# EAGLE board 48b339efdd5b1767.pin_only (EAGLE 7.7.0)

Size 17.78 x 52.07 mm. Coordinates in mm from the lower left corner, seen from the top.
Outline: 0,0 0,52.07 17.78,52.07 17.78,0 0,0
Copper layers (1*16): Top 0.035mm / dielectric 1.5mm / Bottom 0.035mm
Design rules "SparkFun-2-layer-FAB-LIMIT *": minimum track width 4mil, minimum drill 6mil, track to track 6mil, track to pad 6mil, pad to pad 6mil, via to via 6mil, smd to smd 6mil, copper to edge 4mil, drill to drill 4mil, minimum pad ring 5mil, minimum via ring 5mil, stop-mask expansion 4mil, vias tented up to drill 25mil, thermal gap 10mil
tRestrict: 2 lines

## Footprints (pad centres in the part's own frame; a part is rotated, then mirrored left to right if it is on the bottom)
0603 = smd 1.1 x 1: 1 -0.85,0; 2 0.85,0
0402 = smd 0.85 x 0.9: 1 -0.58,0; 2 0.58,0
LED-0603 = smd 1 x 1: A -0.877,0; C 0.877,0
TRACE_ANTENNA_2.4GHZ_15.2MM = smd 0.5 x 0.5: ANT 0,-0.25 | smd 0.9 x 0.5: GND -2.1,-0.25
FIDUCIAL-MICRO = smd 0.635 x 0.635: 1 0,0
1X06 = drill 1.016 pad 1.88: 1 0,0; 2 2.54,0; 3 5.08,0; 4 7.62,0; 5 10.16,0; 6 12.7,0
1X02 = drill 1.016 pad 1.88: 1 0,0; 2 2.54,0
1X17 = drill 1.016 pad 1.88: 1 0,0; 2 2.54,0; 3 5.08,0; 4 7.62,0; 5 10.16,0; 6 12.7,0; 7 15.24,0; 8 17.78,0; 9 20.32,0; 10 22.86,0; 11 25.4,0; 12 27.94,0; 13 30.48,0; 14 33.02,0; 15 35.56,0; 16 38.1,0; 17 40.64,0
2X5-PTH-1.27MM = drill 0.508 pad 1: 1 -2.54,-0.635; 2 -2.54,0.635; 3 -1.27,-0.635; 4 -1.27,0.635; 5 0,-0.635; 6 0,0.635; 7 1.27,-0.635; 8 1.27,0.635; 9 2.54,-0.635; 10 2.54,0.635
SMT-JUMPER_2_NC_TRACE_SILK = smd 0.635 x 1.27: 1 -0.508,0; 2 0.508,0
SMT-JUMPER_2_NO_SILK = smd 0.635 x 1.27: 1 -0.406,0; 2 0.406,0
PAD-JUMPER-2-NC_BY_TRACE_YES_SILK = smd 0.635 x 1.27: 1 -0.508,0; 2 0.508,0
TACTILE_SWITCH_SMD_4.6X2.8MM = smd 0.9 x 1: 1 -2.05,-0.8; 2 2.05,-0.8; 3 2.05,0.8; 4 -2.05,0.8
PAD.03X.04 = smd 1.016 x 1.016: P$1 0,0
SOT23-5 = smd 0.55 x 1.2: 1 -0.95,-1.3; 2 0,-1.3; 3 0.95,-1.3; 4 0.95,1.3; 5 -0.95,1.3
QFN48-6X6MM = smd 0.68 x 0.23: 1 -2.86,2.2; 2 -2.86,1.8; 3 -2.86,1.4; 4 -2.86,1; 5 -2.86,0.6; 6 -2.86,0.2; 7 -2.86,-0.2; 8 -2.86,-0.6; 9 -2.86,-1; 10 -2.86,-1.4; 11 -2.86,-1.8; 12 -2.86,-2.2; 25 2.86,-2.2; 26 2.86,-1.8; 27 2.86,-1.4; 28 2.86,-1; 29 2.86,-0.6; 30 2.86,-0.2; 31 2.86,0.2; 32 2.86,0.6; 33 2.86,1; 34 2.86,1.4; 35 2.86,1.8; 36 2.86,2.2 | smd 0.23 x 0.68: 13 -2.2,-2.86; 14 -1.8,-2.86; 15 -1.4,-2.86; 16 -1,-2.86; 17 -0.6,-2.86; 18 -0.2,-2.86; 19 0.2,-2.86; 20 0.6,-2.86; 21 1,-2.86; 22 1.4,-2.86; 23 1.8,-2.86; 24 2.2,-2.86; 37 2.2,2.86; 38 1.8,2.86; 39 1.4,2.86; 40 1,2.86; 41 0.6,2.86; 42 0.2,2.86; 43 -0.2,2.86; 44 -0.6,2.86; 45 -1,2.86; 46 -1.4,2.86; 47 -1.8,2.86; 48 -2.2,2.86 | smd 4.6 x 4.6: EP 0,0
CRYSTAL-SMD-2.0X1.6MM = smd 0.75 x 0.7: 1 -0.675,-0.5; 2 0.675,-0.5; 3 0.675,0.5; 4 -0.675,0.5
CRYSTAL-SMD-3.2X1.5MM = smd 1 x 1.8: P$1 -1.25,0; P$2 1.25,0

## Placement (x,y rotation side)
C1  1.0uF  [0603]  5.71,6.35 270 top
C2  2.2uF  [0603]  12.06,6.35 270 top
C3  0.1uF  [0402]  6.35,30.48 90 top
C4  DNP  [0402]  7.87,41.91 270 top
C5  100pF  [0402]  6.5,41.91 270 top
C6  1.0uF  [0402]  5.08,33.66 270 top
C7  180pF  [0603]  5.71,24.13 90 top
C8  180pF  [0603]  12.7,24.13 90 top
C9  6pF  [0402]  4.45,43.18 180 top
C10  6pF  [0402]  4.45,39.47 180 top
C11  0.8pF  [0402]  9.53,40.31 0 top
C12  DNP  [0402]  9.53,44.45 180 top
C13  15pF  [0402]  8.13,29.84 180 top
C14  15pF  [0402]  10.59,29.84 0 top
C15  0.1uF  [0402]  13.97,32.77 270 top
C16  0.1uF  [0402]  4.45,38.1 180 top
C17  4.7uF  [0603]  5.08,30.48 270 top
D1  RED  [LED-0603]  6.35,16.51 0 top
D2  BLUE  [LED-0603]  11.43,16.51 0 top
E1  ANT  [TRACE_ANTENNA_2.4GHZ_15.2MM]  4.45,46.99 0 top
FD1  FIDUCIALUFIDUCIAL  [FIDUCIAL-MICRO]  13.59,3.17 0 top
FD2  FIDUCIALUFIDUCIAL  [FIDUCIAL-MICRO]  0.89,46.35 0 top
FRAME1  FRAME-LETTER  [CREATIVE_COMMONS]  not placed on the board
J1  [1X06]  2.54,1.27 0 top
J2  [1X02]  10.16,25.4 180 top
J3  [1X17]  1.27,3.81 90 top
J4  [1X17]  16.51,3.81 90 top
J5  CORTEX_DEBUGPTH  [2X5-PTH-1.27MM]  8.89,19.56 0 top
JP1  VDD-EN  [SMT-JUMPER_2_NC_TRACE_SILK]  8.89,5.71 0 bottom
JP2  NFC1  [SMT-JUMPER_2_NO_SILK]  7.62,23.5 180 bottom
JP3  NFC2  [SMT-JUMPER_2_NO_SILK]  10.16,23.5 0 bottom
JP4  XL1  [PAD-JUMPER-2-NC_BY_TRACE_YES_SILK]  7.62,27.94 180 bottom
JP5  XL2  [PAD-JUMPER-2-NC_BY_TRACE_YES_SILK]  10.16,27.94 0 bottom
JP6  PWR-LED  [PAD-JUMPER-2-NC_BY_TRACE_YES_SILK]  8.89,15.24 0 bottom
L1  3.9nH  [0402]  10.11,42.55 270 top
LOGO1  OSHW-LOGOMINI  [OSHW-LOGO-MINI]  8.89,14.35 0 top
LOGO2  SFE_LOGO_NAME.1_INCH  [SFE_LOGO_NAME_.1]  2.92,48.26 0 top
LOGO3  SFE_LOGO_NAME.1_INCH  [SFE_LOGO_NAME_.1]  14.86,48.26 0 bottom
R1  1k  [0603]  11.43,15.24 0 top
R2  1k  [0603]  6.35,15.24 0 top
SW1  TACTILE_SWITCH_SMD_4_6X2_8MM  [TACTILE_SWITCH_SMD_4.6X2.8MM]  6.35,11.43 90 top
SW2  TACTILE_SWITCH_SMD_4_6X2_8MM  [TACTILE_SWITCH_SMD_4.6X2.8MM]  11.43,11.43 90 top
TP1  TEST-POINT3X4  [PAD.03X.04]  7.62,21.69 0 bottom
TP2  TEST-POINT3X4  [PAD.03X.04]  10.16,21.69 0 bottom
U1  AP2112K-3.3V  [SOT23-5]  8.89,6.35 270 top
U2  NRF52832  [QFN48-6X6MM]  9.53,35.56 90 top
Y1  32MHz  [CRYSTAL-SMD-2.0X1.6MM]  4.45,41.27 90 top
Y2  32.768kHz  [CRYSTAL-SMD-3.2X1.5MM]  8.89,27.94 180 top

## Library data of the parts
C1 = SparkFun-Capacitors; PROD_ID: CAP-00868
C2 = SparkFun-Capacitors; PROD_ID: CAP-07888
C3 C15 C16 = SparkFun-Capacitors; PROD_ID: CAP-12416
C4 C12 = SparkFun-Passives
C5 = nrf52832-breakout-temp; PROD_ID: CAP-13458
C6 = SparkFun-Capacitors; PROD_ID: CAP-12417
C7 C8 = nrf52832-breakout-temp; PROD_ID: CAP-11661
C9 C10 = nrf52832-breakout-temp; PROD_ID: CAP-13455
C11 = nrf52832-breakout-temp; PROD_ID: CAP-13456
C13 C14 = SparkFun-Capacitors; PROD_ID: CAP-13063
C17 = SparkFun-Capacitors; PROD_ID: CAP-08280
D1 = SparkFun-LED; PROD_ID: DIO-00819
D2 = SparkFun-LED; PROD_ID: DIO-08575
E1 = SparkFun-RF
FD1 FD2 FRAME1 LOGO1-LOGO3 = SparkFun-Aesthetics
J1-J5 TP1 TP2 = SparkFun-Connectors
JP1-JP6 = SparkFun-Jumpers
L1 = nrf52832-breakout-temp; PROD_ID: NDUC-13457
R1 R2 = SparkFun-Resistors; PROD_ID: RES-07856
SW1 SW2 = SparkFun-Electromechanical; PROD_ID: SWCH-13065
U1 = SparkFun-PowerIC; PROD_ID: VREG-12457
U2 = nrf52832-breakout-temp; PROD_ID: IC-13460
Y1 = nrf52832-breakout-temp; PROD_ID: XTAL-13459
Y2 = SparkFun-Clocks; PROD_ID: XTAL-13062

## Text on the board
Bottom: v10
tPlace: nRF52832 Breakout | 16 | 15 | 17 | 14 | 18 | 13 | 19 | 12 | 20 | 11 | 22 | 10 | 23 | 09 | 24 | 08 | 25 | 1 | NFC | 2 | 05 / !A3 | 28 / !A4 | 04 / !A2 | 29 / !A5 | 03 / !A1 | 30 / !A6 | PWR | 07 | 02 / !A0 | 31 / !A7 | 01 / !X2 | !RST! | 06 | 00 / !X1 | 3V3 | 3V3 | VIN | VIN | GND | 27 / !TX | 26 / !RX | VCC | GND | GRN | BLK
bPlace: nRF52832 Breakout | http://sfe.io/t549 | 16 | 15 | 17 | 14 | 18 | 13 | 19 | 12 | 20 | 11 | 22 | 10 / !NFC2 | 23 | RTC-EN | 09 / !NFC1 | 24 | 08 | 1 | 2 | 25 | 05 / !A3 | 28 / !A4 | D | C | 04 / !A2 | 29 / !A5 | 03 / !A1 | 30 / !A6 | 02 / !A0 | PWR-LED | 31 / !A7 | 01 / !X2 | !RST! | 00 / !X1 | 3.3V | 3.3V | FTDI / VCC-EN | VIN | VIN | GND | 27 / !TX | 26 / !RX | VCC | GND
Measures: Units in inches
tDocu: Jim Lindblom

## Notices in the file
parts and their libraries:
SparkFun-Aesthetics: Licensing: Creative Commons ShareAlike 4.0 International - https://creativecommons.org/licenses/by-sa/4.0
SparkFun-Aesthetics: Released under the Creative Commons Attribution Share-Alike 4.0 License
SparkFun-Aesthetics: https://creativecommons.org/licenses/by-sa/4.0
